FUNCTION "TAVOLA 2" : VOID
TITLE =TAVOLE DI SOLLEVAMENTO
AUTHOR : LD
FAMILY : DESTECK
NAME : TAVOLA
VERSION : 0.1

BEGIN
NETWORK
TITLE =Tavola 2: Antischiacciamento in corso
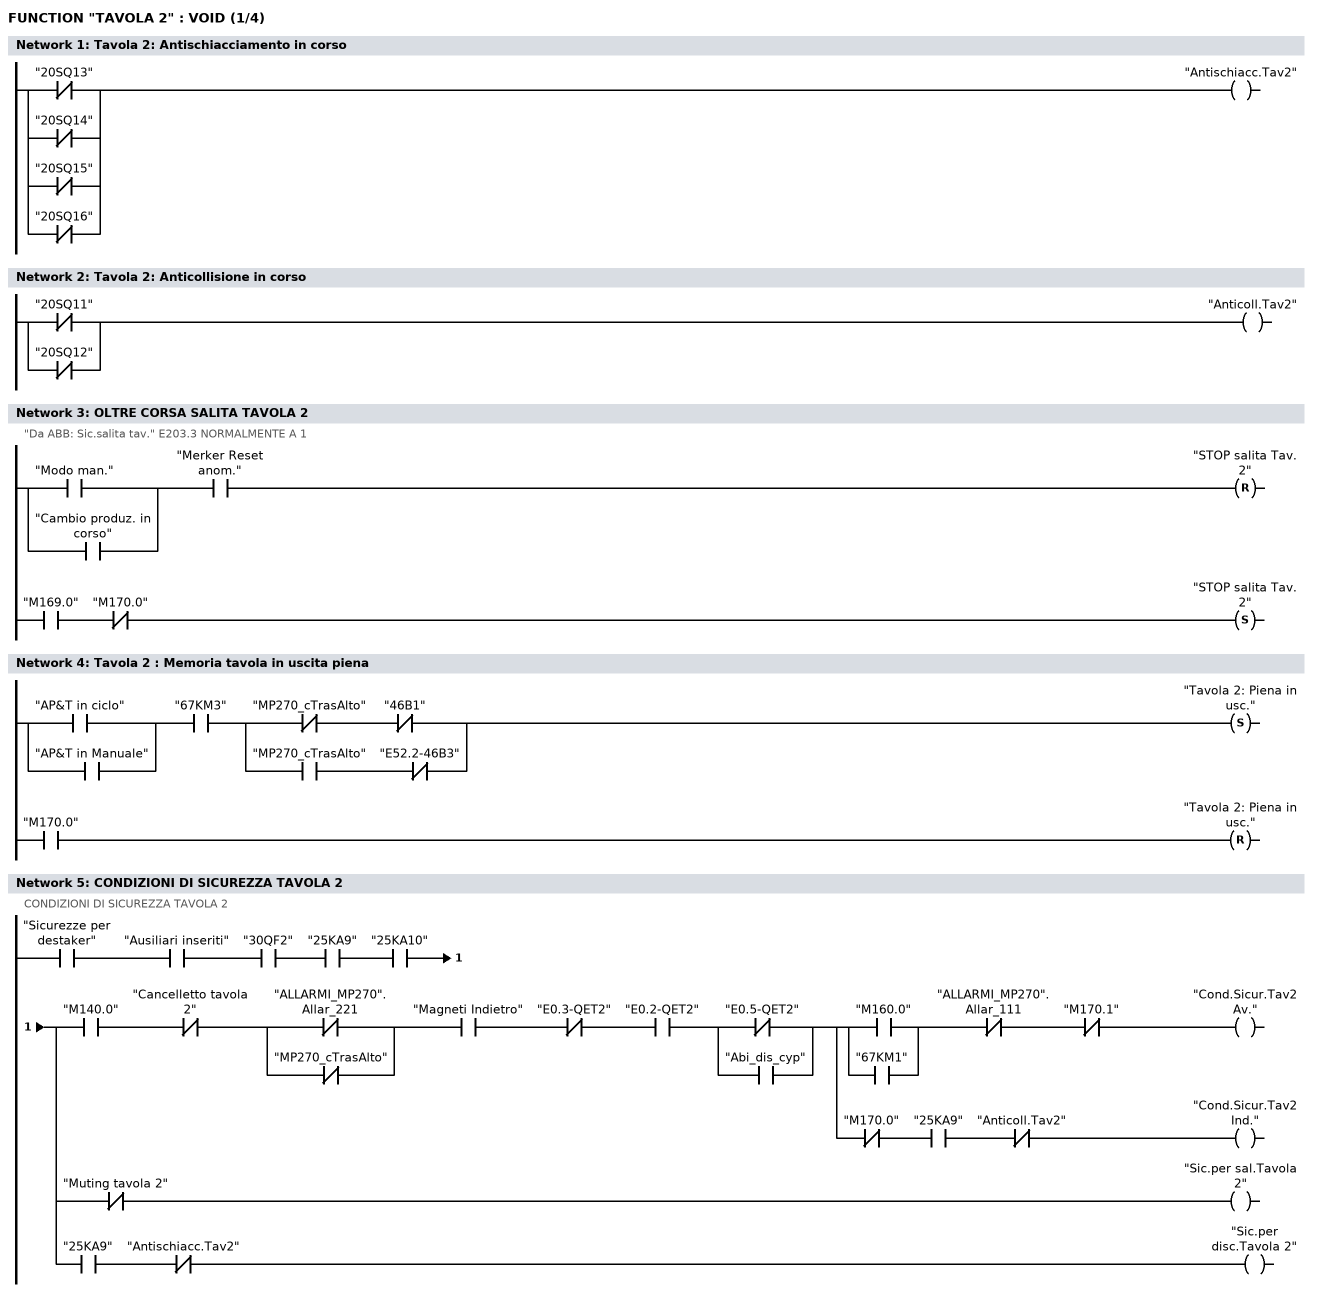
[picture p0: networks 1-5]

      ON    "20SQ13";
      ON    "20SQ14";
      ON    "20SQ15";
      ON    "20SQ16";
      =     "Antischiacc.Tav2";
NETWORK
TITLE =Tavola 2: Anticollisione in corso

      ON    "20SQ11";
      ON    "20SQ12";
      =     "Anticoll.Tav2";
NETWORK
TITLE =OLTRE CORSA SALITA TAVOLA 2
//"Da ABB: Sic.salita tav." E203.3 NORMALMENTE A 1
      U(    ;
      O     "Modo man.";
      O     "Cambio produz. in corso";
      )     ;
      U     "Merker Reset anom.";
      R     "STOP salita Tav. 2";
      U     "M169.0";
      UN    "M170.0";
      S     "STOP salita Tav. 2";
      NOP   0;
NETWORK
TITLE =Tavola 2 : Memoria tavola in uscita piena

      U(    ;
      O     "AP&T  in ciclo";
      O     "AP&T in Manuale";
      )     ;
      U     "67KM3";
      U(    ;
      UN    "MP270_cTrasAlto";
      UN    "46B1";
      O     ;
      U     "MP270_cTrasAlto";
      UN    "E52.2-46B3";
      )     ;
      S     "Tavola 2: Piena in usc.";
      U     "M170.0";
      R     "Tavola 2: Piena in usc.";
      NOP   0;
NETWORK
TITLE =CONDIZIONI DI SICUREZZA TAVOLA 2
//CONDIZIONI DI SICUREZZA TAVOLA 2
      U     "Sicurezze per destaker";
      U     "Ausiliari inseriti";
      U     "30QF2";
      U     "25KA9";
      U     "25KA10";
      =     L      0.0;
      U     L      0.0;
      U     "M140.0";
      UN    "Cancelletto tavola 2";
      U(    ;
      ON    "ALLARMI_MP270".Allar_221;
      ON    "MP270_cTrasAlto";
      )     ;
      U     "Magneti Indietro";
      UN    "E0.3-QET2";
      U     "E0.2-QET2";
      U(    ;
      ON    "E0.5-QET2";
      O     "Abi_dis_cyp";
      )     ;
      =     L      0.1;
      U     L      0.1;
      U(    ;
      O     "M160.0";
      O     "67KM1";
      )     ;
      UN    "ALLARMI_MP270".Allar_111;
      UN    "M170.1";
      =     "Cond.Sicur.Tav2 Av.";
      U     L      0.1;
      UN    "M170.0";
      U     "25KA9";
      UN    "Anticoll.Tav2";
      =     "Cond.Sicur.Tav2 Ind.";
      U     L      0.0;
      UN    "Muting tavola 2";
      =     "Sic.per sal.Tavola 2";
      U     L      0.0;
      U     "25KA9";
      UN    "Antischiacc.Tav2";
      =     "Sic.per disc.Tavola 2";
NETWORK
TITLE =MEMORIA QUOTA RAGGIUNTA TAVOLA 2
//MEMORIA QUOTA RAGGIUNTA TAVOLA 2
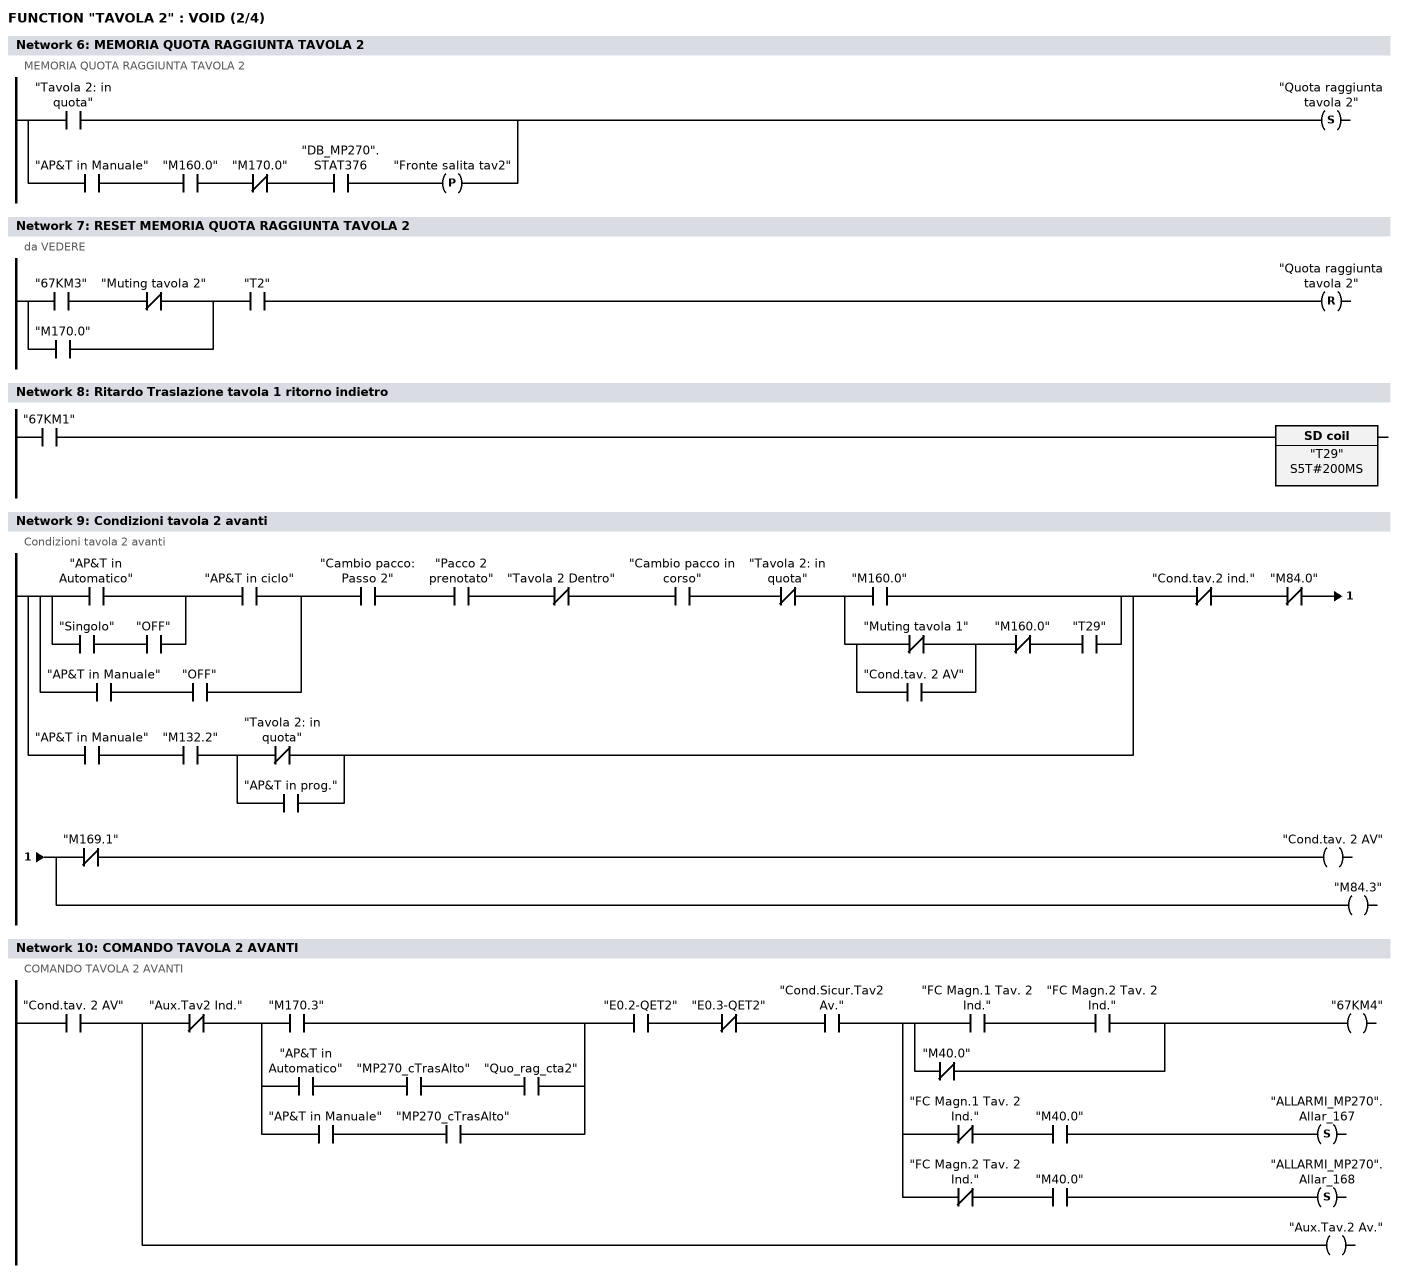
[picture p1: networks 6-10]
      O     "Tavola 2: in quota";
      O(    ;
      U     "AP&T in Manuale";
      U     "M160.0";
      UN    "M170.0";
      U     "DB_MP270".STAT376;
      FP    "Fronte salita tav2";
      )     ;
      S     "Quota raggiunta tavola 2";
NETWORK
TITLE =RESET MEMORIA QUOTA RAGGIUNTA TAVOLA 2
//da VEDERE
      U(    ;
      U     "67KM3";
      UN    "Muting tavola 2";
      O     "M170.0";
      )     ;
      U     "T2";
      R     "Quota raggiunta tavola 2";
NETWORK
TITLE =Ritardo Traslazione tavola 1 ritorno indietro

      U     "67KM1";
      L     S5T#200MS;
      SE    "T29";
NETWORK
TITLE =Condizioni tavola 2 avanti
//Condizioni tavola 2 avanti
      U(    ;
      U(    ;
      U(    ;
      O     "AP&T in Automatico";
      O     ;
      U     "Singolo";
      U     "OFF";
      )     ;
      U     "AP&T  in ciclo";
      O     ;
      U     "AP&T in Manuale";
      U     "OFF";
      )     ;
      U     "Cambio pacco: Passo 2";
      U     "Pacco 2 prenotato";
      UN    "Tavola 2 Dentro";
      U     "Cambio pacco in corso";
      UN    "Tavola 2: in quota";
      U(    ;
      O     "M160.0";
      O     ;
      U(    ;
      ON    "Muting tavola 1";
      O     "Cond.tav. 2  AV";
      )     ;
      UN    "M160.0";
      U     "T29";
      )     ;
      O     ;
      U     "AP&T in Manuale";
      U     "M132.2";
      U(    ;
      ON    "Tavola 2: in quota";
      O     "AP&T in prog.";
      )     ;
      )     ;
      UN    "Cond.tav.2 ind.";
      UN    "M84.0";
      =     L      0.0;
      U     L      0.0;
      UN    "M169.1";
      =     "Cond.tav. 2  AV";
      U     L      0.0;
      BLD   102;
      =     "M84.3";
NETWORK
TITLE = COMANDO TAVOLA 2 AVANTI
// COMANDO TAVOLA 2 AVANTI
      U     "Cond.tav. 2  AV";
      =     L      0.0;
      U     L      0.0;
      UN    "Aux.Tav2 Ind.";
      U(    ;
      O     "M170.3";
      O     ;
      U     "AP&T in Automatico";
      U     "MP270_cTrasAlto";
      U     "Quo_rag_cta2";
      O     ;
      U     "AP&T in Manuale";
      U     "MP270_cTrasAlto";
      )     ;
      U     "E0.2-QET2";
      UN    "E0.3-QET2";
      U     "Cond.Sicur.Tav2 Av.";
      =     L      0.1;
      U     L      0.1;
      U(    ;
      U     "FC Magn.1 Tav. 2 Ind.";
      U     "FC Magn.2 Tav. 2 Ind.";
      ON    "M40.0";
      )     ;
      =     "67KM4";
      U     L      0.1;
      UN    "FC Magn.1 Tav. 2 Ind.";
      U     "M40.0";
      S     "ALLARMI_MP270".Allar_167;
      U     L      0.1;
      UN    "FC Magn.2 Tav. 2 Ind.";
      U     "M40.0";
      S     "ALLARMI_MP270".Allar_168;
      U     L      0.0;
      BLD   102;
      =     "Aux.Tav.2 Av.";
NETWORK
TITLE =Condizioni tavola 2 indietro
//Condizioni tavola 2 indietro
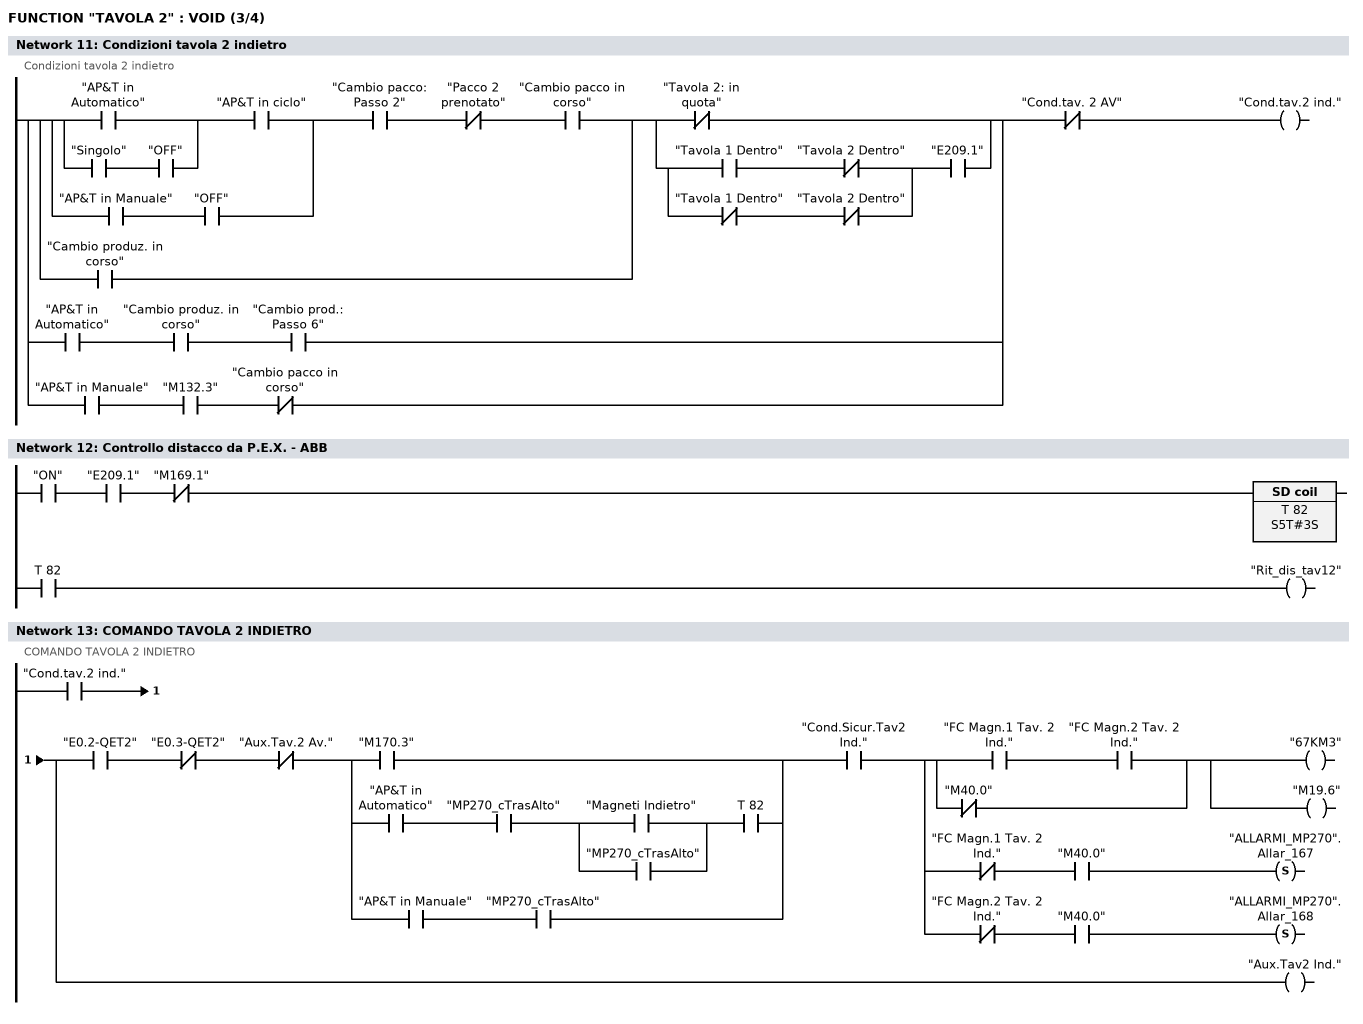
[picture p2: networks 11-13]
      U(    ;
      U(    ;
      U(    ;
      U(    ;
      O     "AP&T in Automatico";
      O     ;
      U     "Singolo";
      U     "OFF";
      )     ;
      U     "AP&T  in ciclo";
      O     ;
      U     "AP&T in Manuale";
      U     "OFF";
      )     ;
      U     "Cambio pacco: Passo 2";
      UN    "Pacco 2 prenotato";
      U     "Cambio pacco in corso";
      O     "Cambio produz. in corso";
      )     ;
      U(    ;
      ON    "Tavola 2: in quota";
      O     ;
      U(    ;
      U     "Tavola 1 Dentro";
      UN    "Tavola 2 Dentro";
      O     ;
      UN    "Tavola 1 Dentro";
      UN    "Tavola 2 Dentro";
      )     ;
      U     "E209.1";
      )     ;
      O     ;
      U     "AP&T in Automatico";
      U     "Cambio produz. in corso";
      U     "Cambio prod.: Passo 6";
      O     ;
      U     "AP&T in Manuale";
      U     "M132.3";
      UN    "Cambio pacco in corso";
      )     ;
      UN    "Cond.tav. 2  AV";
      =     "Cond.tav.2 ind.";
NETWORK
TITLE =Controllo distacco da P.E.X. - ABB

      U     "ON";
      U     "E209.1";
      UN    "M169.1";
      L     S5T#3S;
      SE    T     82;
      NOP   0;
      NOP   0;
      NOP   0;
      U     T     82;
      =     "Rit_dis_tav12";
NETWORK
TITLE =COMANDO TAVOLA 2 INDIETRO
//COMANDO TAVOLA 2 INDIETRO
      U     "Cond.tav.2 ind.";
      =     L      0.0;
      U     L      0.0;
      U     "E0.2-QET2";
      UN    "E0.3-QET2";
      UN    "Aux.Tav.2 Av.";
      U(    ;
      O     "M170.3";
      O     ;
      U     "AP&T in Automatico";
      U     "MP270_cTrasAlto";
      U(    ;
      O     "Magneti Indietro";
      O     "MP270_cTrasAlto";
      )     ;
      U     T     82;
      O     ;
      U     "AP&T in Manuale";
      U     "MP270_cTrasAlto";
      )     ;
      U     "Cond.Sicur.Tav2 Ind.";
      =     L      0.1;
      U     L      0.1;
      U(    ;
      U     "FC Magn.1 Tav. 2 Ind.";
      U     "FC Magn.2 Tav. 2 Ind.";
      ON    "M40.0";
      )     ;
      =     "67KM3";
      =     "M19.6";
      U     L      0.1;
      UN    "FC Magn.1 Tav. 2 Ind.";
      U     "M40.0";
      S     "ALLARMI_MP270".Allar_167;
      U     L      0.1;
      UN    "FC Magn.2 Tav. 2 Ind.";
      U     "M40.0";
      S     "ALLARMI_MP270".Allar_168;
      U     L      0.0;
      BLD   102;
      =     "Aux.Tav2 Ind.";
NETWORK
TITLE =Condizioni salita tavola 2
//Condizioni salita tavola 2
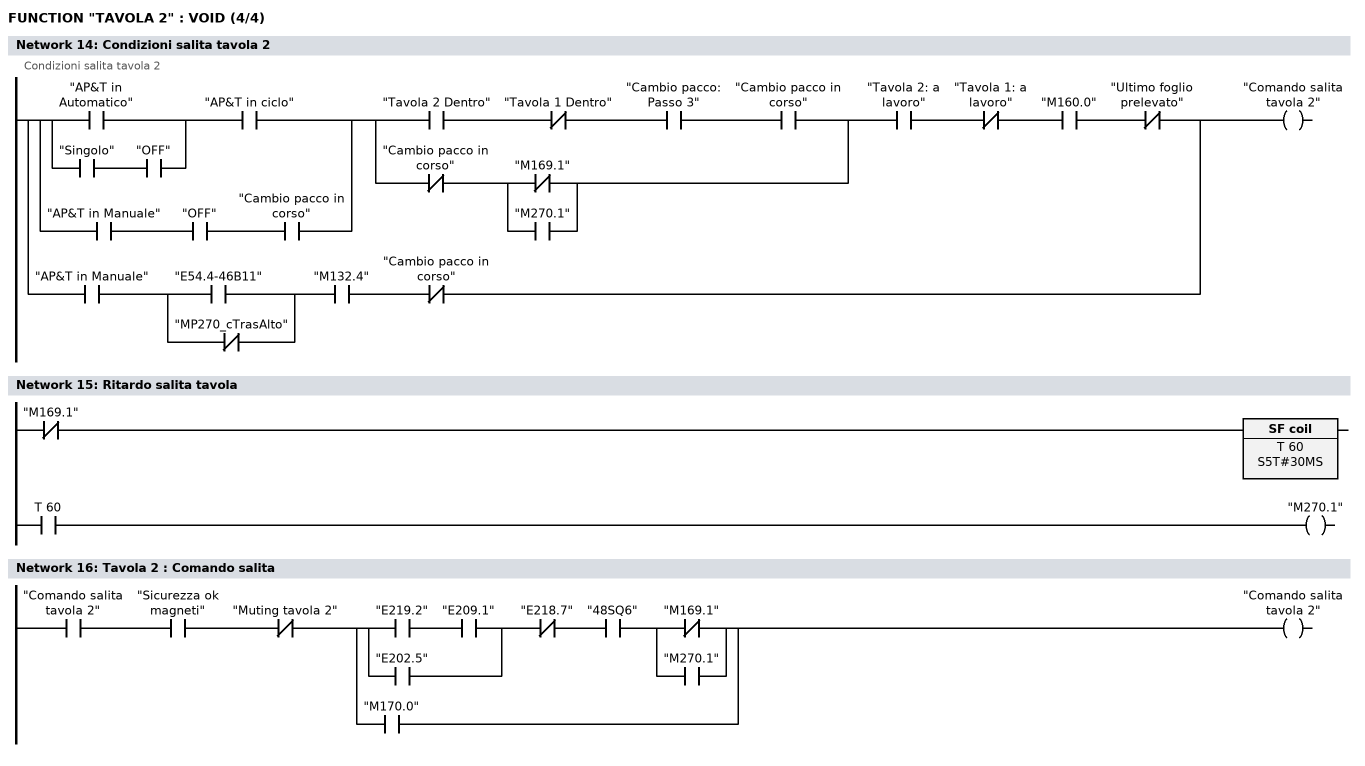
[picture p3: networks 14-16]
      U(    ;
      U(    ;
      O     "AP&T in Automatico";
      O     ;
      U     "Singolo";
      U     "OFF";
      )     ;
      U     "AP&T  in ciclo";
      O     ;
      U     "AP&T in Manuale";
      U     "OFF";
      U     "Cambio pacco in corso";
      )     ;
      U(    ;
      U     "Tavola 2 Dentro";
      UN    "Tavola 1 Dentro";
      U     "Cambio pacco: Passo 3";
      U     "Cambio pacco in corso";
      O     ;
      UN    "Cambio pacco in corso";
      U(    ;
      ON    "M169.1";
      O     "M270.1";
      )     ;
      )     ;
      U     "Tavola 2: a  lavoro";
      UN    "Tavola 1: a  lavoro";
      U     "M160.0";
      UN    "Ultimo foglio prelevato";
      O     ;
      U     "AP&T in Manuale";
      U(    ;
      O     "E54.4-46B11";
      ON    "MP270_cTrasAlto";
      )     ;
      U     "M132.4";
      UN    "Cambio pacco in corso";
      =     "Comando salita tavola 2";
NETWORK
TITLE =Ritardo salita tavola

      UN    "M169.1";
      L     S5T#30MS;
      SA    T     60;
      NOP   0;
      NOP   0;
      NOP   0;
      U     T     60;
      =     "M270.1";
NETWORK
TITLE =Tavola 2 : Comando salita

      U     "Comando salita tavola 2";
      U     "Sicurezza ok magneti";
      UN    "Muting tavola 2";
      U(    ;
      U(    ;
      U     "E219.2";
      U     "E209.1";
      O     "E202.5";
      )     ;
      UN    "E218.7";
      U     "48SQ6";
      U(    ;
      ON    "M169.1";
      O     "M270.1";
      )     ;
      O     "M170.0";
      )     ;
      =     "Comando salita tavola 2";
NETWORK
TITLE =COMANDO SALITA TAVOLA 2
//COMANDO SALITA TAVOLA 2
//MaxZub20101018: ins. condizione per sollevamanto ritardato in cambio pacchi
      U(    ;
      U     "Comando salita tavola 2";
      UN    "Cambio pacco in corso";
      O(    ;
      U     "Comando salita tavola 2";
      U     "Cambio pacco in corso";
      L     S5T#2S;
      SE    "T44";
      NOP   0;
      NOP   0;
      NOP   0;
      U     "T44";
      )     ;
      O     ;
      U     "AP&T in Automatico";
      U     "MP270_cTrasAlto";
      U     "M170.0";
      U     "Mem_sal_pan2";
      )     ;
      U     "Sic.per sal.Tavola 2";
      UN    "STOP salita Tav. 2";
      U     "48SQ3";
      =     "79YV1A";
NETWORK
TITLE =Condizioni discesa tavola 2
//Condizioni discesa tavola 2
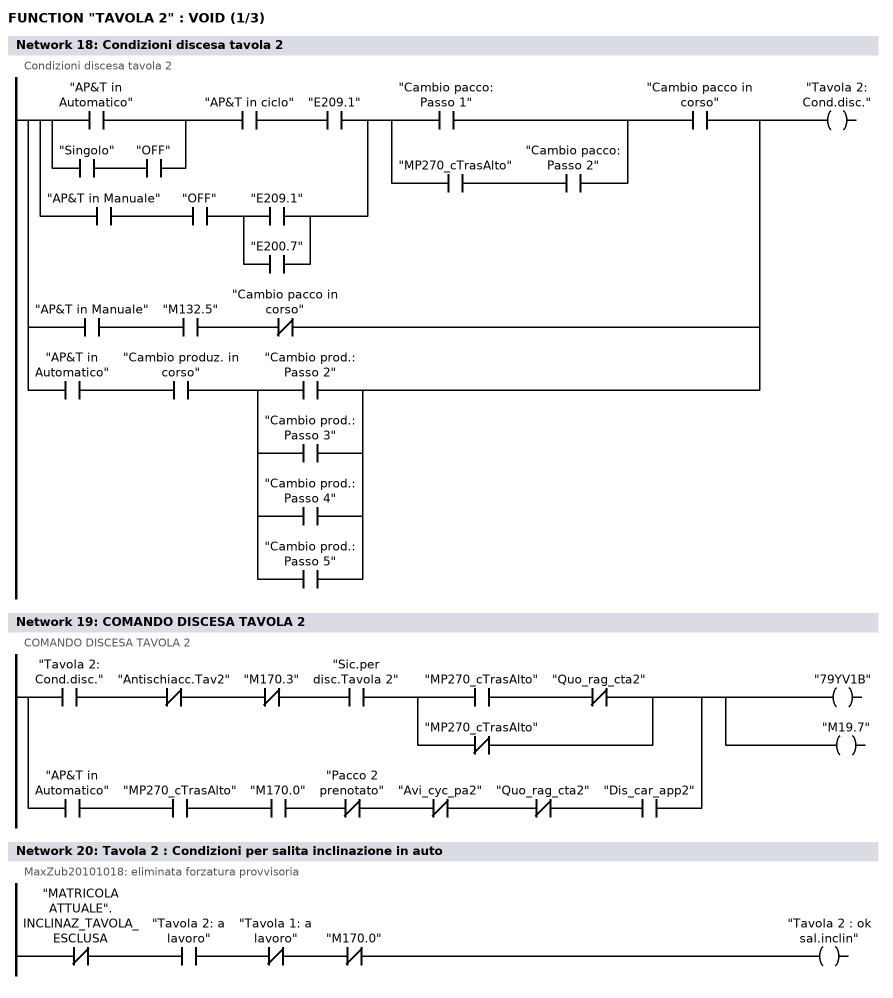
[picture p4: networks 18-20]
      U(    ;
      U(    ;
      O     "AP&T in Automatico";
      O     ;
      U     "Singolo";
      U     "OFF";
      )     ;
      U     "AP&T  in ciclo";
      U     "E209.1";
      O     ;
      U     "AP&T in Manuale";
      U     "OFF";
      U(    ;
      O     "E209.1";
      O     "E200.7";
      )     ;
      )     ;
      U(    ;
      O     "Cambio pacco: Passo 1";
      O     ;
      U     "MP270_cTrasAlto";
      U     "Cambio pacco: Passo 2";
      )     ;
      U     "Cambio pacco in corso";
      O     ;
      U     "AP&T in Manuale";
      U     "M132.5";
      UN    "Cambio pacco in corso";
      O     ;
      U     "AP&T in Automatico";
      U     "Cambio produz. in corso";
      U(    ;
      O     "Cambio prod.: Passo 2";
      O     "Cambio prod.: Passo 3";
      O     "Cambio prod.: Passo 4";
      O     "Cambio prod.: Passo 5";
      )     ;
      =     "Tavola 2: Cond.disc.";
NETWORK
TITLE =COMANDO DISCESA TAVOLA 2
//COMANDO DISCESA TAVOLA 2
      U     "Tavola 2: Cond.disc.";
      UN    "Antischiacc.Tav2";
      UN    "M170.3";
      U     "Sic.per disc.Tavola 2";
      U(    ;
      U     "MP270_cTrasAlto";
      UN    "Quo_rag_cta2";
      ON    "MP270_cTrasAlto";
      )     ;
      O     ;
      U     "AP&T in Automatico";
      U     "MP270_cTrasAlto";
      U     "M170.0";
      UN    "Pacco 2 prenotato";
      UN    "Avi_cyc_pa2";
      UN    "Quo_rag_cta2";
      U     "Dis_car_app2";
      =     "79YV1B";
      =     "M19.7";
NETWORK
TITLE =Tavola 2 : Condizioni per salita inclinazione in auto
//MaxZub20101018: eliminata forzatura provvisoria
      UN    "MATRICOLA ATTUALE".INCLINAZ_TAVOLA_ESCLUSA;
      U     "Tavola 2: a  lavoro";
      UN    "Tavola 1: a  lavoro";
      UN    "M170.0";
      =     "Tavola 2 : ok sal.inclin";
NETWORK
TITLE =Inclinazione tavola 2 sollevamento su
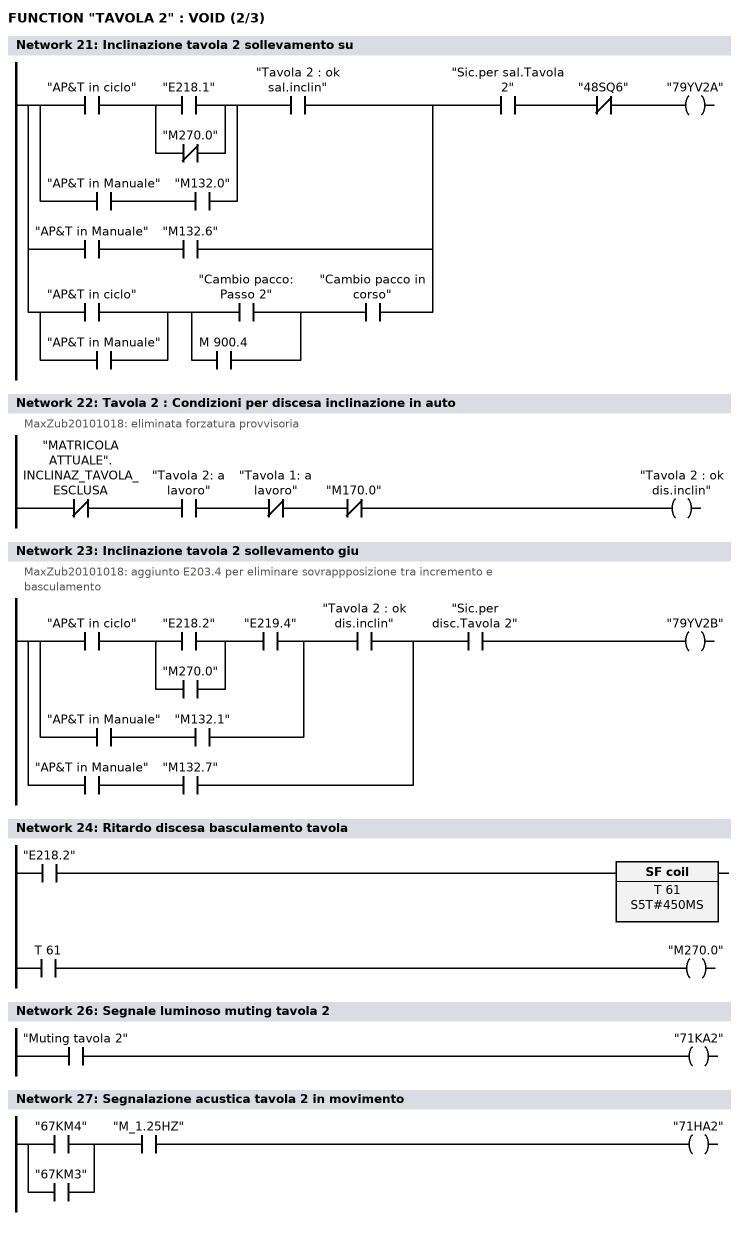
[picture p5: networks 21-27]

      U(    ;
      U(    ;
      U     "AP&T  in ciclo";
      U(    ;
      O     "E218.1";
      ON    "M270.0";
      )     ;
      O     ;
      U     "AP&T in Manuale";
      U     "M132.0";
      )     ;
      U     "Tavola 2 : ok sal.inclin";
      O     ;
      U     "AP&T in Manuale";
      U     "M132.6";
      O     ;
      U(    ;
      O     "AP&T  in ciclo";
      O     "AP&T in Manuale";
      )     ;
      U(    ;
      O     "Cambio pacco: Passo 2";
      O     M    900.4;
      )     ;
      U     "Cambio pacco in corso";
      )     ;
      U     "Sic.per sal.Tavola 2";
      UN    "48SQ6";
      =     "79YV2A";
NETWORK
TITLE =Tavola 2 : Condizioni per discesa inclinazione in auto
//MaxZub20101018: eliminata forzatura provvisoria
      UN    "MATRICOLA ATTUALE".INCLINAZ_TAVOLA_ESCLUSA;
      U     "Tavola 2: a  lavoro";
      UN    "Tavola 1: a  lavoro";
      UN    "M170.0";
      =     "Tavola 2 : ok dis.inclin";
NETWORK
TITLE =Inclinazione tavola 2 sollevamento giu
//MaxZub20101018: aggiunto E203.4 per eliminare sovrappposizione tra incremento e
//basculamento
      U(    ;
      U(    ;
      U     "AP&T  in ciclo";
      U(    ;
      O     "E218.2";
      O     "M270.0";
      )     ;
      U     "E219.4";
      O     ;
      U     "AP&T in Manuale";
      U     "M132.1";
      )     ;
      U     "Tavola 2 : ok dis.inclin";
      O     ;
      U     "AP&T in Manuale";
      U     "M132.7";
      )     ;
      U     "Sic.per disc.Tavola 2";
      =     "79YV2B";
NETWORK
TITLE =Ritardo discesa basculamento tavola

      U     "E218.2";
      L     S5T#450MS;
      SA    T     61;
      NOP   0;
      NOP   0;
      NOP   0;
      U     T     61;
      =     "M270.0";
NETWORK
TITLE =

NETWORK
TITLE =Segnale luminoso muting tavola 2

      U     "Muting tavola 2";
      =     "71KA2";
NETWORK
TITLE =Segnalazione acustica tavola 2 in movimento

      U(    ;
      O     "67KM4";
      O     "67KM3";
      )     ;
      U     "M_1.25HZ";
      =     "71HA2";
NETWORK
TITLE =COMANDO POMPA TAVOLA 2
//COMANDO POMPA TAVOLA 2
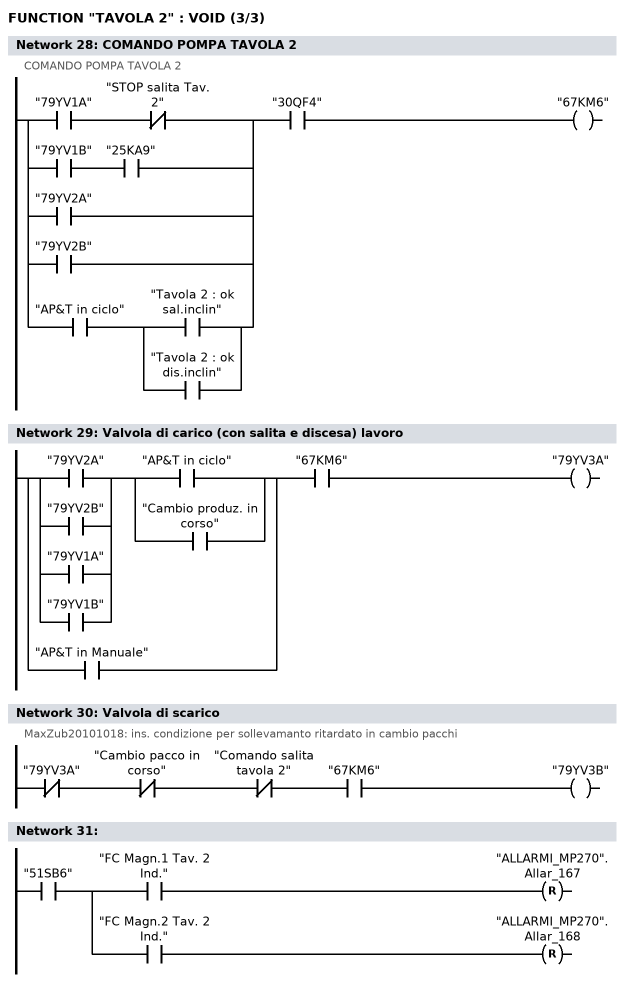
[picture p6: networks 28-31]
      U(    ;
      U     "79YV1A";
      UN    "STOP salita Tav. 2";
      O     ;
      U     "79YV1B";
      U     "25KA9";
      O     "79YV2A";
      O     "79YV2B";
      O     ;
      U     "AP&T  in ciclo";
      U(    ;
      O     "Tavola 2 : ok sal.inclin";
      O     "Tavola 2 : ok dis.inclin";
      )     ;
      )     ;
      U     "30QF4";
      =     "67KM6";
NETWORK
TITLE =Valvola di carico (con salita e discesa) lavoro

      U(    ;
      U(    ;
      O     "79YV2A";
      O     "79YV2B";
      O     "79YV1A";
      O     "79YV1B";
      )     ;
      U(    ;
      O     "AP&T  in ciclo";
      O     "Cambio produz. in corso";
      )     ;
      O     "AP&T in Manuale";
      )     ;
      U     "67KM6";
      =     "79YV3A";
NETWORK
TITLE =Valvola di scarico
//MaxZub20101018: ins. condizione per sollevamanto ritardato in cambio pacchi
      UN    "79YV3A";
      UN    "Cambio pacco in corso";
      UN    "Comando salita tavola 2";
      U     "67KM6";
      =     "79YV3B";
NETWORK
TITLE =

      U     "51SB6";
      =     L      0.0;
      U     L      0.0;
      U     "FC Magn.1 Tav. 2 Ind.";
      R     "ALLARMI_MP270".Allar_167;
      U     L      0.0;
      U     "FC Magn.2 Tav. 2 Ind.";
      R     "ALLARMI_MP270".Allar_168;
END_FUNCTION

